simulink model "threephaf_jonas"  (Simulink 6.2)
settings: Solver=ode23  StartTime=0  StopTime=0.05  FixedStep=0.000001  MaxStep=2e-5  RelTol=1e-3
undefined symbols (not defined in the file or in its folder): Cdc, di, DiscIntNeverNeededParam, Element, L, R, Symmetrized, Tf, Ts, Udc, Upp, Warning, Yes
libraries: simulink x12
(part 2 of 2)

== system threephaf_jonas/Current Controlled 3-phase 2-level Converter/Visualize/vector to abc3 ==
  vect : Inport  Port=1  LatchInput=off
  Ü> a : Fcn  Expr=sqrt(2/3)*u[1]
  Ü> b : Fcn  Expr=-sqrt(1/6)*u[1]+sqrt(1/2)*u[2]
  Ü> c : Fcn  Expr=-sqrt(1/6)*u[1]-sqrt(1/2)*u[2]
  a : Outport  InitialOutput=0
  b : Outport  Port=2  InitialOutput=0
  c : Outport  Port=3  InitialOutput=0
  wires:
  Ü> a/1 -> a/1
  Ü> c/1 -> c/1
  Ü> b/1 -> b/1
  vect/1 -> Ü> c/1, Ü> a/1, Ü> b/1

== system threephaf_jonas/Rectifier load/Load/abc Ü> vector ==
  a : Inport  Port=1  LatchInput=off
  b : Inport  Port=2  LatchInput=off
  c : Inport  Port=3  LatchInput=off
  Fcn : Fcn  Expr=sqrt(3/2)*u[1]
  Fcn1 : Fcn  Expr=sqrt(1/2)*(u[1]-u[2])
  Gain : Gain  Gain=1/3
  Mux5 : Mux  Inputs=2
  Mux7 : Mux  Inputs=2
  Sum2 : Sum  Inputs=+++
  Ü> ua : Sum  Inputs=+-
  Ü> ub : Sum  Inputs=+-
  Ü> uc : Sum  Inputs=+-
  vect : Outport  InitialOutput=0
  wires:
  c/1 -> Sum2/3, Ü> uc/1
  Sum2/1 -> Gain/1
  b/1 -> Sum2/2, Ü> ub/1
  a/1 -> Sum2/1, Ü> ua/1
  Gain/1 -> Ü> ua/2, Ü> ub/2, Ü> uc/2
  Ü> ua/1 -> Fcn/1
  Ü> ub/1 -> Mux7/1
  Ü> uc/1 -> Mux7/2
  Mux7/1 -> Fcn1/1
  Mux5/1 -> vect/1
  Fcn/1 -> Mux5/1
  Fcn1/1 -> Mux5/2

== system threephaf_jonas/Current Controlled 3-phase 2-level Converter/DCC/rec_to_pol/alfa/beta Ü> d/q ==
  vect : Inport  Port=1  LatchInput=off
  angle : Inport  Port=2  LatchInput=off
  Fcn : Fcn  Expr=u[1]*cos(u[3])-u[2]*sin(u[3])
  Fcn1 : Fcn  Expr=u[1]*sin(u[3])+u[2]*cos(u[3])
  Mux : Mux  Inputs=2
  Mux1 : Mux  Inputs=2
  Out : Outport  InitialOutput=0
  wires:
  vect/1 -> Mux/1
  angle/1 -> Mux/2
  Mux/1 -> Fcn/1, Fcn1/1
  Fcn/1 -> Mux1/1
  Fcn1/1 -> Mux1/2
  Mux1/1 -> Out/1

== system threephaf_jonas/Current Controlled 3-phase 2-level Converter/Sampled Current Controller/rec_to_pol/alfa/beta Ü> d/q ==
  vect : Inport  Port=1  LatchInput=off
  angle : Inport  Port=2  LatchInput=off
  Fcn : Fcn  Expr=u[1]*cos(u[3])-u[2]*sin(u[3])
  Fcn1 : Fcn  Expr=u[1]*sin(u[3])+u[2]*cos(u[3])
  Mux : Mux  Inputs=2
  Mux1 : Mux  Inputs=2
  Out : Outport  InitialOutput=0
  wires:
  vect/1 -> Mux/1
  angle/1 -> Mux/2
  Mux/1 -> Fcn/1, Fcn1/1
  Fcn/1 -> Mux1/1
  Fcn1/1 -> Mux1/2
  Mux1/1 -> Out/1
